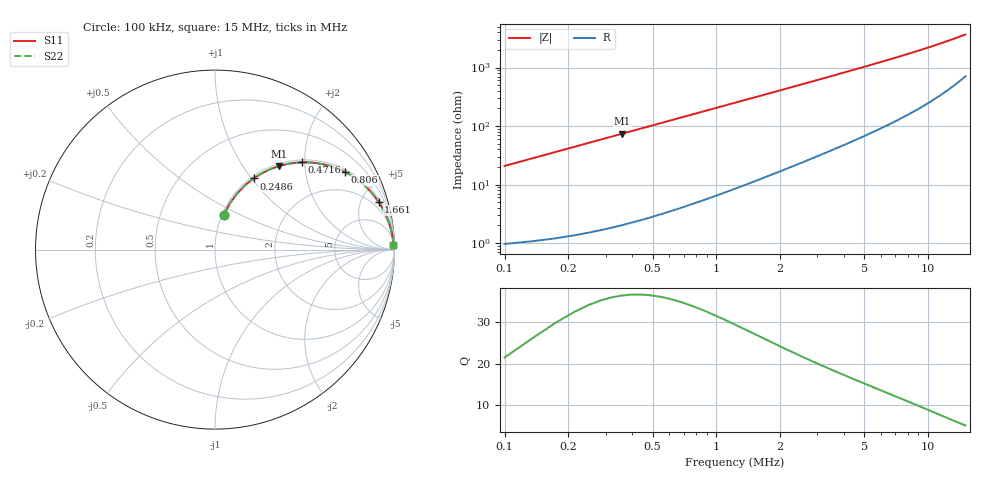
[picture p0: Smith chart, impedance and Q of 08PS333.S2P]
! Coilcraft 0805PS-333 Power Chip Inductor
! 5 February 2003
# MHZ S MA R 50
!Freq  MagS11  AngS11  MagS21  AngS21  MagS12  AngS12  MagS22  AngS22
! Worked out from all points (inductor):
!   402 points, 100 kHz to 15 MHz, reference 50 ohm
!   read as one part in series: L = 32.8 uH near 174.3 kHz
!   highest Q = 36.4 at 360.1 kHz (marker M1), where L = 32.7 uH
!   S11 on the Smith chart (normalised r, x): 100 kHz: 1.02, +0.41; 248.6 kHz: 1.03, +1.02; 471.6 kHz: 1.05, +1.93; 806 kHz: 1.10, +3.29; 1.661 MHz: 1.26, +6.76; 15 MHz: 15, +72
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0.1  0.2015 75.7  0.9702 -11.6  0.9702 -11.6  0.2015 75.7
0.17432  0.3355 68.5  0.9309 -19.6  0.9309 -19.6  0.3355 68.5
0.21148  0.3956 64.9  0.9063 -23.3  0.9063 -23.3  0.3956 64.9
0.24864  0.4508 61.5  0.8795 -26.8  0.8795 -26.8  0.4508 61.5
0.2858  0.5011 58.3  0.8514 -30.1  0.8514 -30.1  0.5011 58.3
0.36012  0.5874 52.5  0.7934 -36.0  0.7934 -36.0  0.5874 52.5
0.4716  0.686 45.1  0.7091 -43.3  0.7091 -43.3  0.686 45.1
0.62024  0.7751 37.6  0.6104 -50.8  0.6104 -50.8  0.7751 37.6
0.80604  0.8438 30.8  0.5122 -57.5  0.5122 -57.5  0.8438 30.8
0.99184  0.8855 25.9  0.4374 -62.3  0.4374 -62.3  0.8855 25.9
1.17764  0.9124 22.3  0.38 -65.8  0.38 -65.8  0.9124 22.3
1.4006  0.9334 19.1  0.3271 -68.9  0.3271 -68.9  0.9334 19.1
1.66072  0.9491 16.3  0.2807 -71.5  0.2807 -71.5  0.9491 16.3
2.10664  0.9649 13.0  0.2251 -74.6  0.2251 -74.6  0.9649 13.0
2.58972  0.9742 10.6  0.1848 -76.7  0.1848 -76.7  0.9742 10.6
3.70452  0.9843 7.5  0.1301 -79.4  0.1301 -79.4  0.9843 7.5
5.07944  0.9893 5.4  0.09453 -80.8  0.09453 -80.8  0.9893 5.4
6.2314  0.9913 4.4  0.07642 -81.3  0.07642 -81.3  0.9913 4.4
7.56916  0.9927 3.5  0.06204 -81.5  0.06204 -81.5  0.9927 3.5
10.05888  0.9939 2.6  0.045 -81.0  0.045 -81.0  0.9939 2.6
12.5486  0.9944 1.9  0.03434 -79.6  0.03434 -79.6  0.9944 1.9
15  0.9944 1.5  0.02707 -77.4  0.02707 -77.4  0.9944 1.5
